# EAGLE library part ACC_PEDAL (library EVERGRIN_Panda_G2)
Accelerator pedal
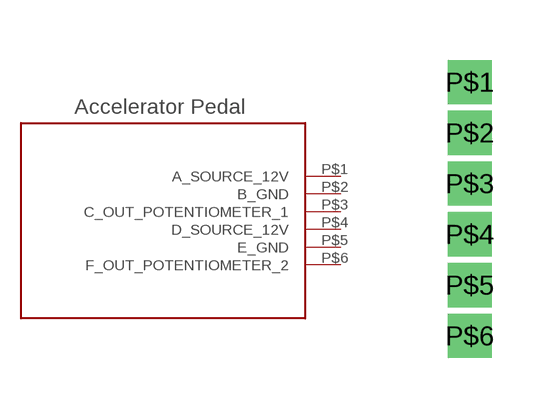
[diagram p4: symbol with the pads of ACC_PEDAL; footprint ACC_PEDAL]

Designator prefix -

## ACC_PEDAL  [ACC_PEDAL]
P$1  A_SOURCE_12V
P$2  B_GND
P$3  C_OUT_POTENTIOMETER_1
P$4  D_SOURCE_12V
P$5  E_GND
P$6  F_OUT_POTENTIOMETER_2

## Footprint ACC_PEDAL (pad centres in mm)
drill 0.6 square: P$1 5.08,11.43; P$2 5.08,10.16; P$3 5.08,8.89; P$4 5.08,7.62; P$5 5.08,6.35; P$6 5.08,5.08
